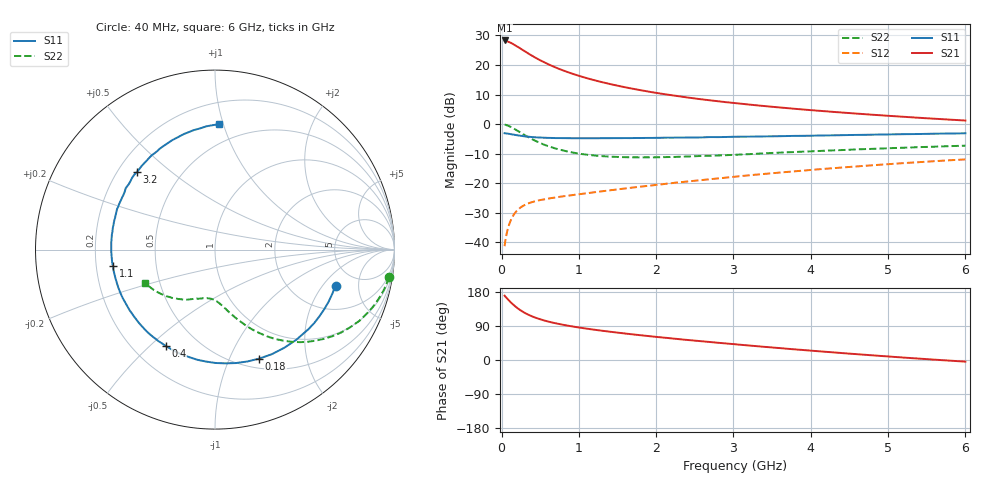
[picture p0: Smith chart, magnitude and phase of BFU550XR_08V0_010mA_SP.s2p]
! Filename:  P:\Prog\Test\Noise\ATS_data\Testdata_Net\03 Spar\BFU550XR_APG2013_45_C05_08p0V_010mA_SP_CM01_D.s2p
! Date/Time: Tue 06/Aug/2013 14:38:17
! BFU550XR_APG2013_45_C05_08p0V_1to35mA_SP_CM01_Bias5_R.s2p
! MDIF S-parameter v. bias file
! BFU550XR_APG2013_45_C05_08p0V_1to35mA_SP_CM01
! Date/time Fri Aug 02 14:53:20 2013
! VAR V_out= 8.0000
! VAR I_out= 9.9900
! VAR V_in= 0.8127
! VAR I_in= 0.1061
! Device data file deembeded for feedlines and parallel
! Original file: \03 Spar\BFU550XR_APG2013_45_C05_08p0V_010mA_SP_CM01_R.s2p
! Feed-files: PR006V01_02082013_Feed1.s2p, PR006V01_02082013_Feed2.s2p
! Parallel-file: PR006V01_02082013_Par.s2p
# MHz S MA R 50
!  Freq-MHz  S11-mag  S11-arg  S21-mag  S21-arg  S12-mag  S12-arg  S22-mag  S22-arg
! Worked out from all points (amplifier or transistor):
!   98 points, 40 MHz to 6 GHz, reference 50 ohm
!   highest |S21| = 28.3 dB at 40 MHz (marker M1)
!   |S21| within 3 dB of that: start of sweep to 260.5 MHz
!   unconditionally stable (mu >= 1): 1.936 GHz to 3.921 GHz
!   at 300 MHz: K = 0.28, MSG = 26.0 dB, |S12| = -27.4 dB
!   at 1.6 GHz: K = 0.94, MSG = 17.1 dB, |S12| = -21.8 dB
!   at 6 GHz: K = 0.87, MSG = 6.6 dB, |S12| = -11.9 dB
!   S11 on the Smith chart (normalised r, x): 40 MHz: 3.45, -2.71; 180 MHz: 0.61, -1.30; 400 MHz: 0.33, -0.56; 1.1 GHz: 0.27, -0.07; 3.2 GHz: 0.28, +0.39; 6 GHz: 0.35, +0.97
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40  0.7014 -16.6  26.06 169.8  0.008601 81.7  0.9793 -9.0
50  0.6984 -20.6  25.93 166.9  0.01072 80.4  0.9746 -11.4
80  0.6902 -32.7  25.01 160.6  0.01662 74.8  0.9454 -18.1
120  0.6765 -47.9  23.78 152.1  0.02362 68.2  0.8971 -26.2
140  0.6693 -54.8  23.02 148.2  0.02668 65.3  0.8682 -29.9
180  0.6553 -67.9  21.44 141.1  0.03209 60.0  0.8109 -36.6
220  0.6427 -79.6  19.97 134.8  0.03638 55.9  0.7544 -42.3
280  0.626 -94.3  17.77 126.8  0.04141 51.0  0.6762 -49.6
340  0.6138 -106.8  15.88 120.3  0.04512 47.4  0.6088 -55.3
400  0.6029 -117.0  14.25 114.8  0.04806 44.9  0.5524 -59.9
500  0.5935 -130.2  12.05 107.6  0.05186 42.3  0.48 -65.9
650  0.5834 -144.8  9.704 99.2  0.05618 40.8  0.4048 -72.5
800  0.5799 -155.5  8.08 92.8  0.06007 40.6  0.3574 -77.3
1050  0.5771 -168.6  6.285 84.3  0.06627 41.8  0.3104 -83.4
1100  0.5762 -170.8  6.014 82.8  0.0676 42.1  0.3045 -84.5
1500  0.5792 174.8  4.475 72.2  0.07862 44.3  0.2784 -92.0
2050  0.5868 160.0  3.299 60.0  0.09516 46.4  0.2755 -100.8
3100  0.6134 137.0  2.215 40.1  0.1323 46.7  0.306 -115.5
3200  0.614 134.9  2.146 38.3  0.1361 46.5  0.3101 -116.8
4100  0.6411 118.6  1.686 23.1  0.1719 43.0  0.3506 -129.1
5200  0.676 100.2  1.332 6.4  0.219 36.3  0.399 -143.8
6000  0.6998 88.0  1.151 -4.3  0.2529 30.2  0.432 -154.5
